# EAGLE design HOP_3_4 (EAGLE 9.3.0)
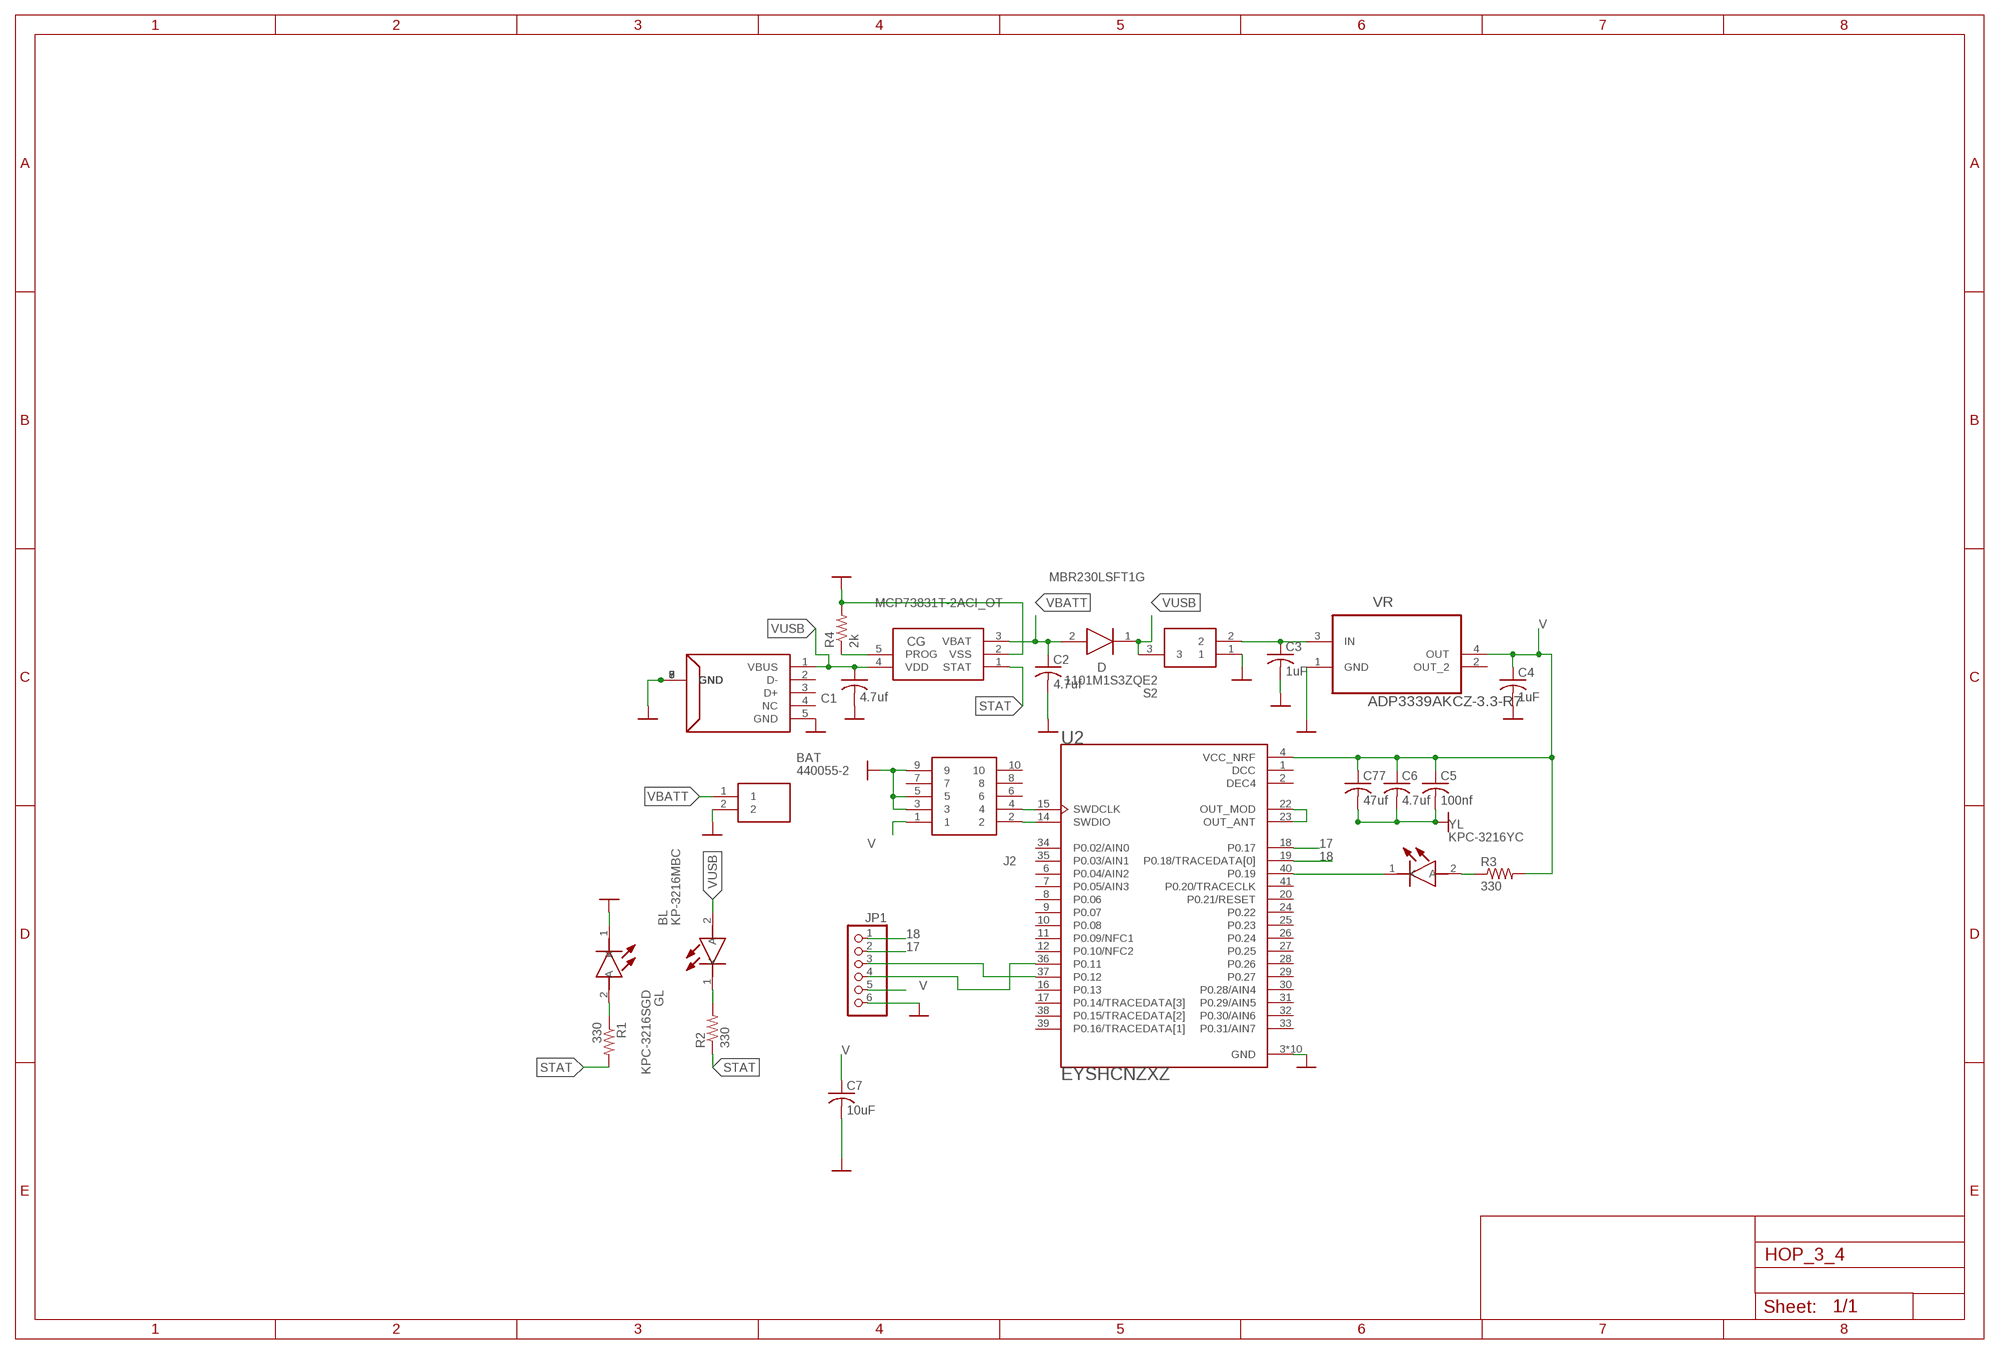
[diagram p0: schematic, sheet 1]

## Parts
BAT  440055-2  [SHDR2W70P0X200_1X2_600X770X525]
BL  KP-3216MBC  [LEDC3216X130N]
C1  4.7uf  C-USC0805  [C0805]
C2  4.7uf  C-USC0805  [C0805]
C3  1uF  C-USC0805  [C0805]
C4  1uF  C-USC0805  [C0805]
C5  100nf  C-USC0805  [C0805]
C6  4.7uf  C-USC0805  [C0805]
C7  10uF  C-USC0805  [C0805]
C77  47uf  C-USC0805  [C0805]
CG  MCP73831T-2ACI_OT  [SOT95P270X145-5N]
D  MBR230LSFT1G  [SODFL3616X98N]
GL  KPC-3216SGD  [LEDC3216X110N]
J2  20021121-00010C4LF  [20021121-00010C4LF]
JP1  PINHD-1X6  [1X06]
R1  330  R-US_R0805  [R0805]
R2  330  R-US_R0805  [R0805]
R3  330  R-US_R0805  [R0805]
R4  2k  R-US_R0805  [R0805]
S2  1101M1S3ZQE2  [1000-SERIES(SPDT)]
U2  EYSHCNZXZ  [XCVR_EYSHCNZXZ]
USB  MC001009  [MC001009]
VR  ADP3339AKCZ-3.3-R7  [SOT230P700X180-4N]
YL  KPC-3216YC  [LEDC3216X110N]

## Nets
17: JP1.2 U2.18(P0.17)
18: JP1.1 U2.19(P0.18/TRACEDATA[0])
GND: BAT.2 C1.2 C2.2 C3.2 C4.2 C5.2 C6.2 C7.2 C77.2 CG.2(VSS) GL.1(K) J2.3 J2.5 J2.9 JP1.6 R4.2 S2.1 U2.3(GND) U2.5(GND) U2.13(GND) U2.21(GND) U2.42(GND) U2.43(GND) U2.44(GND) U2.45(GND) U2.47(GND) U2.48(GND) USB.5(GND) USB.6(GND) USB.7(GND) USB.8(GND) USB.9(GND) VR.1(GND) ; supply symbol labelled GND-BAR
N$1: U2.22(OUT_MOD) U2.23(OUT_ANT)
N$2: CG.5(PROG) R4.1
N$3: BL.1(K) R2.2
N$4: GL.2(A) R1.1
N$5: U2.40(P0.19) YL.1(K)
N$6: J2.4 U2.15(SWDCLK)
N$7: J2.2 U2.14(SWDIO)
N$8: C3.1 S2.2 VR.3(IN)
N$9: R3.1 YL.2(A)
N$10: JP1.3 U2.37(P0.12)
N$11: JP1.4 U2.36(P0.11)
STAT: CG.1(STAT) R1.2 R2.1
V [power]: C4.1 C5.1 C6.1 C7.1 C77.1 J2.1 JP1.5 R3.2 U2.4(VCC_NRF) VR.4(OUT)
VBATT [power]: BAT.1 C2.1 CG.3(VBAT) D.2(A)
VUSB [power]: BL.2(A) C1.1 CG.4(VDD) D.1(K) S2.3 USB.1(VBUS)
Unconnected: J2.6 J2.7 J2.8 J2.10 U2.6(P0.04/AIN2) U2.7(P0.05/AIN3) U2.8(P0.06) U2.9(P0.07) U2.10(P0.08) U2.11(P0.09/NFC1) U2.12(P0.10/NFC2) U2.16(P0.13) U2.17(P0.14/TRACEDATA[3]) U2.20(P0.21/RESET) U2.24(P0.22) U2.25(P0.23) U2.26(P0.24) U2.27(P0.25) U2.28(P0.26) U2.29(P0.27) U2.30(P0.28/AIN4) U2.31(P0.29/AIN5) U2.32(P0.30/AIN6) U2.33(P0.31/AIN7) U2.34(P0.02/AIN0) U2.35(P0.03/AIN1) U2.38(P0.15/TRACEDATA[2]) U2.39(P0.16/TRACEDATA[1]) U2.41(P0.20/TRACECLK) USB.2(D-) USB.3(D+) USB.4(NC) VR.2(OUT_2)

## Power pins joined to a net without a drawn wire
DCC: U2.1(DCC)
DEC4: U2.2(DEC4)

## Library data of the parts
BAT = Battery2mm:440055-2: AMP - TE CONNECTIVITY - 440055-2 - CONNECTOR, HEADER, 2POS, 1ROW, 2MM; DESCRIPTION: AMP - TE CONNECTIVITY - 440055-2 - CONNECTOR, HEADER, 2POS, 1ROW, 2MM; HEIGHT: 5.25mm; MANUFACTURER_NAME: TE Connectivity; MANUFACTURER_PART_NUMBER: 440055-2; MOUSER_PART_NUMBER: 571-440055-2; MOUSER_PRICE-STOCK: https://www.mouser.com/Search/Refine.aspx?Keyword=571-440055-2
BL = blue led:KP-3216MBC: Kingbright KP-3216MBC, 1206 466 nm Blue LED, 3216 (1206) SMD package; DESCRIPTION: Kingbright KP-3216MBC, 1206 466 nm Blue LED, 3216 (1206) SMD package; HEIGHT: 1.3mm; MANUFACTURER_NAME: Kingbright; MANUFACTURER_PART_NUMBER: KP-3216MBC; MOUSER_PART_NUMBER: N/A; MOUSER_PRICE-STOCK: https://www.mouser.com/Search/Refine.aspx?Keyword=N%2FA; RS_PART_NUMBER: 1651739; RS_PRICE-STOCK: http://uk.rs-online.com/web/p/products/1651739
C1-C7 C77 = rcl:C-US: CAPACITOR, American symbol; SPICEPREFIX: C
CG = BCharger:MCP73831T-2ACI_OT: Li-Ion Charge Controller 4.2V SOT23-5 Source: Datasheet; ALLIED_NUMBER: 70046198; ALLIED_PRICE-STOCK: http://www.alliedelec.com/microchip-technology-inc-mcp73831t-2aci-ot/70046198/; DESCRIPTION: Li-Ion Charge Controller 4.2V SOT23-5; HEIGHT: 1.45mm; MANUFACTURER_NAME: Microchip; MANUFACTURER_PART_NUMBER: MCP73831T-2ACI/OT; MOUSER_PART_NUMBER: 579-MCP73831T-2ACIOT; MOUSER_PRICE-STOCK: https://www.mouser.com/Search/Refine.aspx?Keyword=579-MCP73831T-2ACIOT; RS_PART_NUMBER: 2508396481; RS_PRICE-STOCK: http://uk.rs-online.com/web/p/products/2508396481
D = Schttoky diode:MBR230LSFT1G: Diode Schottky 30V 2A SOD123FL ON Semiconductor MBR230LSFT1G Schottky Diode, 2A, 30V, 2-Pin SOD-123FL; ALLIED_NUMBER: 70300366; ALLIED_PRICE-STOCK: http://www.alliedelec.com/on-semiconductor-mbr230lsft1g/70300366/; DESCRIPTION: Diode Schottky 30V 2A SOD123FL ON Semiconductor MBR230LSFT1G Schottky Diode, 2A, 30V, 2-Pin SOD-123FL; HEIGHT: 0.98mm; MANUFACTURER_NAME: ON Semiconductor; MANUFACTURER_PART_NUMBER: MBR230LSFT1G; MOUSER_PART_NUMBER: 863-MBR230LSFT1G; MOUSER_PRICE-STOCK: https://www.mouser.com/Search/Refine.aspx?Keyword=863-MBR230LSFT1G; RS_PART_NUMBER: 1630931; RS_PRICE-STOCK: http://uk.rs-online.com/web/p/products/1630931
GL = Green LED:KPC-3216SGD: KINGBRIGHT - KPC-3216SGD - LED, SMD, 1206, DIFFUSED, GREEN; DESCRIPTION: KINGBRIGHT - KPC-3216SGD - LED, SMD, 1206, DIFFUSED, GREEN; HEIGHT: 1.1mm; MANUFACTURER_NAME: Kingbright; MANUFACTURER_PART_NUMBER: KPC-3216SGD; MOUSER_PART_NUMBER: N/A; MOUSER_PRICE-STOCK: https://www.mouser.com/Search/Refine.aspx?Keyword=N%2FA
J2 = SWD pins:20021121-00010C4LF: Headers & Wire Housings 1.27x1.27mm BTB, Hdr Unshrd, SMT, 10 Pos Source: Datasheet; ALLIED_NUMBER: 70247660; ALLIED_PRICE-STOCK: http://www.alliedelec.com/fci-20021121-00010c4lf/70247660/; DESCRIPTION: Headers & Wire Housings 1.27x1.27mm BTB, Hdr Unshrd, SMT, 10 Pos; HEIGHT: mm; MANUFACTURER_NAME: FCI; MANUFACTURER_PART_NUMBER: 20021121-00010C4LF; MOUSER_PART_NUMBER: 649-202112100010C4LF; MOUSER_PRICE-STOCK: https://www.mouser.com/Search/Refine.aspx?Keyword=649-202112100010C4LF; RS_PART_NUMBER: 1708866; RS_PRICE-STOCK: http://uk.rs-online.com/web/p/products/1708866
JP1 = pinhead:PINHD-1X6: PIN HEADER
R1-R4 = rcl:R-US_: RESISTOR, American symbol; SPICEPREFIX: R
S2 = SSS:1101M1S3ZQE2: 2 position SPDT panel mount slide switch Panel Mount Slide Switch SPDT On-On 6 A@ 120 V ac, 6 A@ 28 V dc Slide Source: Datasheet; ALLIED_NUMBER: 70128206; ALLIED_PRICE-STOCK: https://www.alliedelec.com/c-k-1101m1s3zqe2/70128206/; DESCRIPTION: 2 position SPDT panel mount slide switch Panel Mount Slide Switch SPDT On-On 6 A@ 120 V ac, 6 A@ 28 V dc Slide; HEIGHT: mm; MANUFACTURER_NAME: C & K COMPONENTS; MANUFACTURER_PART_NUMBER: 1101M1S3ZQE2; MOUSER_PART_NUMBER: 611-1101M1S3ZQE2; MOUSER_PRICE-STOCK: https://www.mouser.com/Search/Refine.aspx?Keyword=611-1101M1S3ZQE2; RS_PART_NUMBER: 1617328; RS_PRICE-STOCK: http://uk.rs-online.com/web/p/products/1617328
U2 = My_module:EYSHCNZXZ: Wireless Module: Bluetooth Smart (BLE); DESCRIPTION: Wireless Module: Bluetooth? Smart _BLE_; MP: EYSHCNZXZ
USB = USB:MC001009
VR = Analoge_Phase-2:ADP3339AKCZ-3.3-R7: Low Dropout Regulator; MPN: ADP3339AKCZ-3.3-R7; OC_FARNELL: 2112615; OC_NEWARK: 12M8168; PACKAGE: SOT-223-3; SUPPLIER: Analog Devices
YL = yellow led:KPC-3216YC: KINGBRIGHT - KPC-3216YC - LED, SMD, CLR LENS, YELLOW; DESCRIPTION: KINGBRIGHT - KPC-3216YC - LED, SMD, CLR LENS, YELLOW; HEIGHT: 1.1mm; MANUFACTURER_NAME: Kingbright; MANUFACTURER_PART_NUMBER: KPC-3216YC; MOUSER_PART_NUMBER: N/A; MOUSER_PRICE-STOCK: https://www.mouser.com/Search/Refine.aspx?Keyword=N%2FA

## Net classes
0 default: width 0.15 mm, drill 0.254 mm, clearance 0.152 mm
1 power: width 0.5 mm, clearance 0.152 mm

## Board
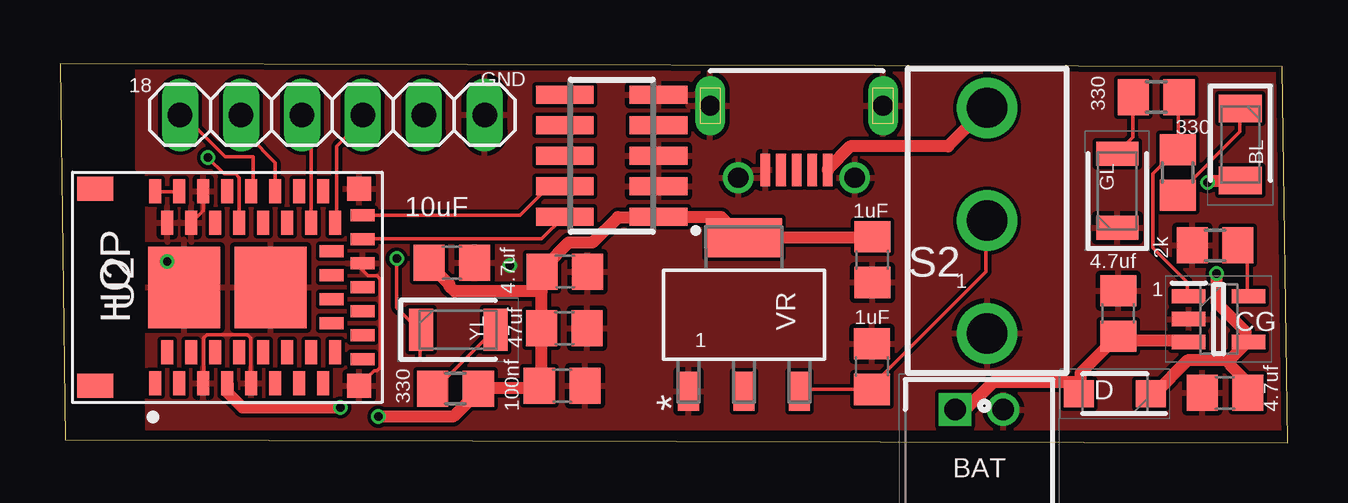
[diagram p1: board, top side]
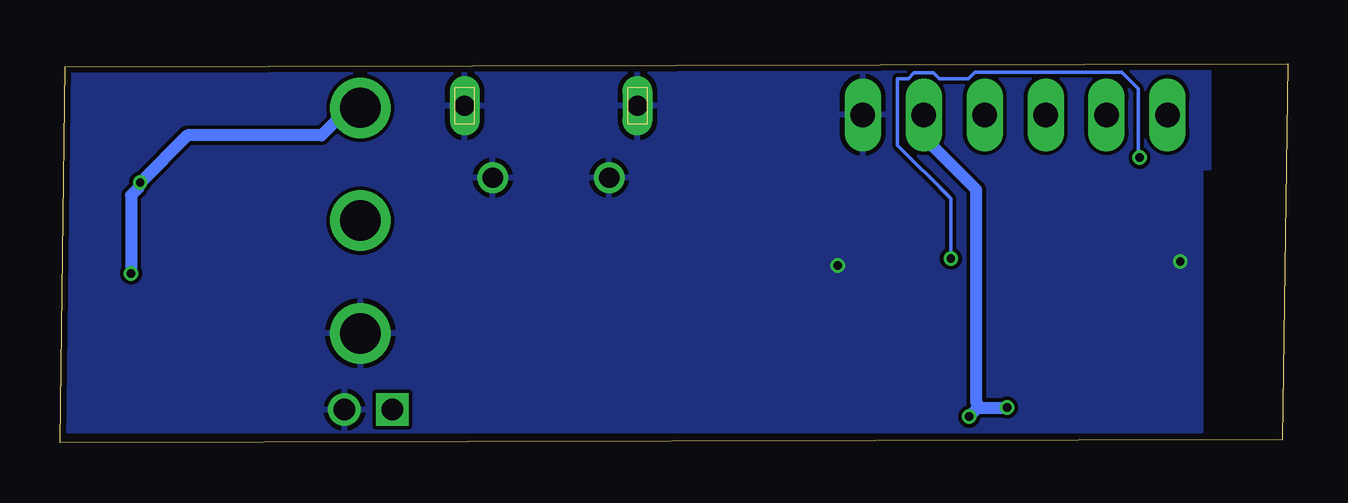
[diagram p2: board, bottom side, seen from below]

Size 51.17 x 15.8 mm. Coordinates in mm from the lower left corner, seen from the top.
Outline: 0.23,0.13 51.17,0 50.94,15.67 0,15.8 0.23,0.13
Copper layers (1*16): Top 0.018mm / dielectric 1.55mm / Bottom 0.018mm
Design rules "eC_2Layer_PClass6_BaseCopperO18_eCDefault": minimum track width 0.15mm, minimum drill 0.35mm, track to track 0.15mm, track to pad 0.15mm, pad to pad 0.15mm, via to via 0.15mm, smd to smd 0mil, copper to edge 0.25mm, drill to drill 0.35mm, minimum pad ring 0.175mm, minimum via ring 0.125mm, stop-mask expansion 0mil, vias tented up to drill 0.45mm, thermal gap 0.2mm

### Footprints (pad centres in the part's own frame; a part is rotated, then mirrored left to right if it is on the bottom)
SHDR2W70P0X200_1X2_600X770X525 = drill 0.9 pad 1.35 square: 1 0,0 | drill 0.9 pad 1.35: 2 2,0
LEDC3216X130N = smd 1.15 x 1.8: 1 -1.5,0; 2 1.5,0
C0805 = smd 1.3 x 1.5: 1 -0.95,0; 2 0.95,0
SOT95P270X145-5N = smd 1.4 x 0.6: 1 -1.25,0.95; 2 -1.25,0; 3 -1.25,-0.95; 4 1.25,-0.95; 5 1.25,0.95
SODFL3616X98N = smd 1.24 x 1.12: 1 -1.5,0; 2 1.5,0
LEDC3216X110N = smd 1 x 1.75: 1 -1.55,0; 2 1.55,0
20021121-00010C4LF = smd 0.76 x 2.4: 1 -2.54,-1.95; 2 -2.54,1.95; 3 -1.27,-1.95; 4 -1.27,1.95; 5 0,-1.95; 6 0,1.95; 7 1.27,-1.95; 8 1.27,1.95; 9 2.54,-1.95; 10 2.54,1.95
1X06 = drill 1.016 long: 1 -6.35,0; 2 -3.81,0; 3 -1.27,0; 4 1.27,0; 5 3.81,0; 6 6.35,0
R0805 = smd 1.3 x 1.5: 1 -0.95,0; 2 0.95,0
1000-SERIES(SPDT) = drill 1.68 pad 2.48: 1 0,-4.7; 2 0,0; 3 0,4.7
XCVR_EYSHCNZXZ = smd 0.5 x 1: 1 -3,-4; 2 -2,-4; 3 -1,-4; 4 0,-4; 5 1,-4; 6 2,-4; 7 3,-4; 8 4,-4; 16 4,4; 17 3,4; 18 2,4; 19 1,4; 20 0,4; 21 -1,4; 22 -2,4; 23 -3,4; 24 -2.5,-2.7; 25 -1.5,-2.7; 26 -0.5,-2.7; 27 0.5,-2.7; 28 1.5,-2.7; 29 2.5,-2.7; 30 3.5,-2.7; 31 4.5,-2.7; 36 4.5,2.7; 37 3.5,2.7; 38 2.5,2.7; 39 1.5,2.7; 40 0.5,2.7; 41 -0.5,2.7; 42 -1.5,2.7; 43 -2.5,2.7 | smd 1 x 0.5: 9 5.65,-3; 10 5.65,-2; 11 5.65,-1; 12 5.65,0; 13 5.65,1; 14 5.65,2; 15 5.65,3; 32 4.35,-1.5; 33 4.35,-0.5; 34 4.35,0.5; 35 4.35,1.5 | smd 3 x 3.4: 44 -1.8,0; 45 1.8,0 | smd 1.5 x 1: 46 -5.5,-4.1; 49 -5.5,4.1 | smd 1 x 1: 47 5.5,-4.1; 48 5.5,4.1
MC001009 = smd 0.4 x 1.35: 1 2.3,2.675; 2 2.95,2.675; 3 3.6,2.675; 4 4.25,2.675; 5 4.9,2.675 | drill 0.83 long: 6 0,0; 7 7.2,0 | drill 0.85: 8 1.175,3; 9 6.025,3
SOT230P700X180-4N = smd 1.626 x 0.889: 1 -3.2,2.311; 2 -3.2,0; 3 -3.2,-2.311 | smd 1.626 x 3.175: 4 3.2,0

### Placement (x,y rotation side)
BAT  37.31,1.38 0 top
BL  49.2,12.43 270 top
C1  48.56,2.08 180 top
C2  44.11,5.38 90 top
C3  33.85,3.17 90 top
C4  33.86,7.63 270 top
C5  20.93,2.37 0 top
C6  21.04,7.14 0 top
C7  16.33,7.51 0 top
C77  21.02,4.78 0 top
CG  48.3,5.16 0 top
D  43.97,2.04 180 top
GL  44.07,10.5 90 top
J2  23,11.96 90 top
JP1  11.35,13.67 0 top
R1  45.69,14.4 0 top
R2  46.58,11.26 270 top
R3  16.48,2.26 0 top
R4  48.15,8.23 180 top
S2  38.65,9.26 0 top
U2  6.97,6.48 0 top
USB  34.3,14.05 180 top
VR  28.51,5.35 90 top
YL  16.6,4.71 0 top

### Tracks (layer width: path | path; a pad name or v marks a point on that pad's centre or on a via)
17
  Top 0.15: U2.18 8.97,10.54 8.97,11.67 7.88,12.76 JP1.2
18
  Top 0.15: U2.19 7.91,10.54 8.05,10.68 8.05,11.91 6.88,11.91 5.13,13.67 JP1.1
GND  (via drill 0.35)
  Top 0.15: U2.21 5.97,9.68 U2.42 | U2.3 5.99,2.5 5.99,4.37 6.13,4.5 7.82,4.5 7.95,4.37 7.95,2.5 U2.5 | U2.13 12.47,7.33 12.84,6.95 13.22,6.95 13.35,6.82 13.35,3.13 13.22,3 13.09,3 U2.47 | U2.44 4.47,7.18 v4.47,7.56
  other vias: 18.76,7.39
  pour Top: 3.62,0.56 3.62,11.39 3.19,11.39 3.19,15.72 50.89,15.72 50.89,0.58
  pour Bottom: 3.58,11.43 3.24,11.43 3.24,15.77 51.03,15.77 51.03,0.47 3.58,0.47
N$1
  Top 0.15: U2.23 3.98,10.46 4.96,10.46 U2.22
N$2
  Top 0.15: CG.5 49.49,6.16 49.49,7.82 49.11,8.2 R4.1
N$3
  Top 0.15: R2.2 46.62,10.39 49.19,12.96 49.19,13.87 BL.1
N$4
  Top 0.15: R1.1 44.73,14.4 44.73,12.73 44.12,12.13 GL.2
N$5  (via drill 0.35)
  Top 0.15: 15.01,4.64 15.01,3.58 | 15.01,4.64 YL.1 | 15.01,4.64 14.03,5.62 v14.03,7.68 | 7.45,8.91 7.45,9.1 U2.40 7.47,11.05 7.32,11.2 6.84,11.2 v6.17,11.88
  Bottom 0.15: v14.03,7.68 14.03,10.17 14.1,10.24 | 14.1,10.24 14.47,10.6 | 14.1,10.24 14.1,10.25 16.26,12.41 16.26,15.18 15.81,15.18 15.57,15.42 14.75,15.42 14.51,15.18 13.3,15.18 13.03,15.44 6.91,15.44 6.22,14.76 6.22,11.94 v6.17,11.88
N$6
  Top 0.15: U2.15 12.67,9.48 19.17,9.48 20.38,10.69 20.99,10.69 J2.4
N$7
  Top 0.15: U2.14 12.67,8.5 20.08,8.5 20.99,9.41 J2.2
N$8
  Top 0.15: VR.3 30.89,2.15 30.97,2.22 C3.1 33.91,2.3 33.91,2.45 38.6,7.14 38.6,9.25 S2.2
N$9
  Top 0.15: R3.1 15.54,2.3 15.69,2.3 18.11,4.72 YL.2
N$10
  Top 0.15: U2.37 10.48,12.73 10.08,13.22 JP1.3
N$11
  Top 0.15: U2.36 11.54,9.18 11.54,12.35 12.61,13.43 JP1.4
STAT
  Top 0.15: CG.1 46.99,6.16 46.99,6.68 45.56,8.12 45.56,11.22 46.54,12.2 R2.1 46.62,12.28 46.62,14.4 R1.2
V  (via drill 0.35)
  Top 0.5: C4.1 33.84,8.57 28.55,8.57 VR.4 28.32,8.65 27.56,9.41 24.99,9.41 J2.1 24.69,9.41 23.25,9.41 22.2,8.35 21.21,8.35 20.23,7.36 C6.1 20.08,7.06 20.08,6.31 | v11.69,1.47 7.61,1.47 7,2.07 7,2.45 U2.4 | v13.28,1.09 16.38,1.09 17.51,2.22 R3.2 17.74,2.3 19.93,2.3 C5.1 20.08,2.6 20.08,4.72 C77.1 20.08,5.02 20.08,6.31 | 20.08,6.31 16.45,6.31 16.22,6.53 16.22,6.61 15.39,7.44 C7.1
  Bottom 0.5: 12.9,1.47 v11.69,1.47 | v13.28,1.09 12.9,1.47 | JP1.5 14.94,13.5 14.94,12.51 12.97,10.54 12.97,1.69 12.9,1.47
VBATT
  Top 0.5: CG.3 46.99,4.27 44.27,4.27 C2.1 44.04,4.42 42.53,2.9 42.53,2.07 D.2 42.31,2.53 38.9,2.53 37.77,1.39 BAT.1
VUSB  (via drill 0.35)
  Top 0.5: 48.73,3.43 46.99,3.43 45.63,2.07 45.48,2.07 D.1 | 48.73,3.43 49.49,4.19 CG.4 49.41,4.42 49.41,4.64 48.2,5.85 v48.2,7.06 | C1.1 49.49,2.15 49.49,2.53 48.81,3.21 48.73,3.43 | USB.1 32.02,11.37 32.02,11.45 32.93,12.35 37.01,12.35 38.6,13.94 S2.3 | v47.82,10.84 47.9,10.92 49.19,10.92 BL.2
  Bottom 0.5: S2.3 38.68,13.94 39.13,13.94 40.26,12.81 45.86,12.81 v47.82,10.84 47.9,10.62 48.2,10.31 v48.2,7.06

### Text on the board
tNames: 18 | GND | 1 | 1 | HOP | 1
